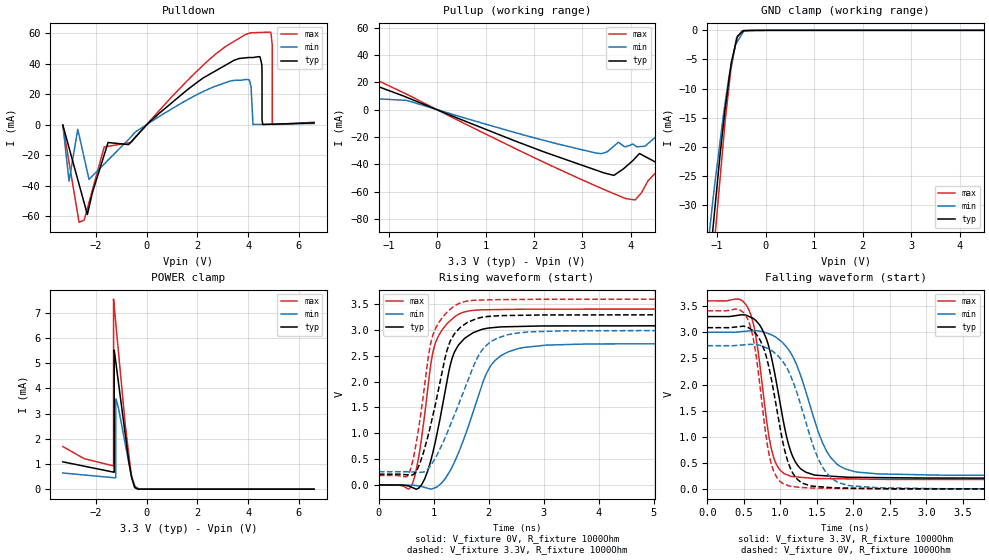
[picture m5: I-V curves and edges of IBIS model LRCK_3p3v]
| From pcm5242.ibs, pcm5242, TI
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|   Model
[Model]   LRCK_3p3v
Model_type   I/O
Polarity   Non-Inverting
Enable   Active-Low
Vinl = 0.99
Vinh = 2.31
Vmeas = 1.65
Vref = 0
Cref = 1pF
Rref = 1000000
|   typ   min   max
C_comp   1.193pF   1.163pF   1.236pF
[Voltage Range]   3.3   3   3.6
[Temperature Range]   27   105   -25
[Pullup Reference]   3.3   3   3.6
[Pulldown Reference]   -0   -0   -0
[Power Clamp Reference]   3.3   3   3.6
[GND Clamp Reference]   -0   -0   -0
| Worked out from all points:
|   slope of the pulldown table from 0 to 0.495 V, typ, clamps not added: 64.7 ohm
|   slope of the pullup table from 0 to 0.495 V, typ, clamps not added: 69.1 ohm
|   GND clamp passes 1 mA (typ) near -0.58 V on its own axis
|   POWER clamp passes 1 mA (typ) near -0.68 V on its own axis
|   falling waveform, V_fixture 3.3V, R_fixture 1000Ohm: 20-80 % time 269ps typ, 407ps min, 199ps max; typ from 3.3 V to 0.207 V
|   rising waveform, V_fixture 0V, R_fixture 1000Ohm: 20-80 % time 359ps typ, 556ps min, 277ps max; typ from 0 V to 3.09 V
|   rising waveform, V_fixture 3.3V, R_fixture 1000Ohm: 20-80 % time 401ps typ, 626ps min, 299ps max; typ from 0.207 V to 3.3 V
|   falling waveform, V_fixture 0V, R_fixture 1000Ohm: 20-80 % time 264ps typ, 397ps min, 195ps max; typ from 3.09 V to 0 V
[Pulldown]
|   Voltage   I(typ)   I(min)   I(max)
-3.3V     -378.6uA   -354.3uA   -383.8uA
-3.055V   -15.23mA   -37.15mA   -24.72mA
-2.66V    -39.19mA   -6.88mA    -64mA
-2.269V   -54.26mA   -35.93mA   -51.02mA
-1.518V   -11.76mA   -23.31mA   -14.25mA
3.893V    43.72mA    29.58mA    58.97mA
4.473V    44.3mA     92.29uA    60.35mA
4.899V    184uA      218.7uA    60.28mA
4.952V    211.8uA    234.3uA    51.71mA
4.954V    212.8uA    234.8uA    45.96mA
4.954V    213uA      234.9uA    123.7nA
6.6V      1.085mA    722.9uA    1.49mA
[GND Clamp]
|   Voltage   I(typ)   I(min)   I(max)
-3.3V     -526.5mA   -489.6mA   -552.8mA
-1.164V   -40.81mA   -35.07mA   -48.1mA
-1.079V   -33.47mA   -28.6mA    -39.08mA
-1.046V   -30.55mA   -26.19mA   -35.49mA
-940.1mV  -21.43mA   -19.22mA   -25.56mA
-837.1mV  -13.61mA   -12.6mA    -15.87mA
-718mV    -6.168mA   -6.453mA   -6.856mA
-600.4mV  -1.708mA   -2.193mA   -1.374mA
-580.8mV  -1.006mA   -1.922mA   -1.157mA
-482.7mV  -273.3uA   -561.9uA   -69.67uA
-284.5mV  -34uA      -2.302uA   -308.8nA
6.6V      0A         0A         0A
[Pullup]
|   Voltage   I(typ)   I(min)   I(max)
-3.3V     20.89mA    12mA       56.35mA
-2.931V   39.44mA    11.28mA    50.14mA
3.451V    -46.27mA   -31.45mA   -58.41mA
4.087V    -35.4mA    -26.27mA   -65.94mA
4.851V    -29.44mA   -9.628mA   -42.22mA
5.092V    -17.54mA   16.01mA    -44.35mA
5.643V    53.42mA    42.85mA    12.66mA
5.844V    57.49mA    46.25mA    45.19mA
6.411V    39.73mA    55.8mA     58.85mA
6.425V    38.25mA    56.04mA    20.59mA
6.504V    29.88mA    -235.4mA   -195.5mA
6.6V      -527.7mA   -587.8mA   -456.8mA
[POWER Clamp]
|   Voltage   I(typ)   I(min)   I(max)
-3.3V     1.085mA    641.9uA    1.693mA
-1.306V   677.2uA    455.6uA    924.8uA
-1.303V   676.5uA    455.2uA    1.01mA
-1.303V   676.5uA    455.2uA    1.69mA
-1.303V   676.4uA    455.2uA    7.179mA
-1.303V   676.4uA    455.2uA    7.549mA
-1.276V   766.2uA    452.7uA    7.258mA
-1.276V   5.221mA    452.7uA    7.257mA
-1.275V   5.526mA    452.7uA    7.255mA
-1.206V   4.992mA    3.578mA    6.509mA
-482.7mV  140.9uA    192.3uA    79.12uA
6.6V      0A         0A         0A
[Ramp]
R_load = 1000
|   typ   min   max
dV/dt_r   1.85276/3.58741e-10   1.64632/5.53781e-10   2.04618/2.76561e-10
dV/dt_f   1.85579/2.6927e-10   1.64679/4.06983e-10   2.05064/1.98632e-10
[Falling Waveform]
V_fixture = 3.3V
V_fixture_min = 3V
V_fixture_max = 3.6V
R_fixture = 1000Ohm
C_fixture = 0F
|   Time   V(typ)   V(min)   V(max)
0s        3.3V       3V         3.6V
565.5ps   3.304V     3.025V     3.437V
675.7ps   3.206V     3.028V     2.818V
830ps     2.78V      2.977V     1.126V
894.2ps   2.411V     2.94V      671.4mV
1.141ns   727.9mV    2.607V     246.7mV
1.287ns   380.2mV    2.135V     226.4mV
1.631ns   253.8mV    730.7mV    201.1mV
2.023ns   226mV      334.4mV    194.4mV
10ns      207mV      255.4mV    182.3mV
[Rising Waveform]
V_fixture = 0V
V_fixture_min = 0V
V_fixture_max = 0V
R_fixture = 1000Ohm
C_fixture = 0F
|   Time   V(typ)   V(min)   V(max)
0s        1.762nV    46.88nV    912.6pV
565.5ps   -31.63mV   -4.28mV    -62.7mV
779.9ps   6.321mV    -32.44mV   929.2mV
939.8ps   450.6mV    -79.6mV    2.294V
1.029ns   844.6mV    -52.35mV   2.748V
1.312ns   2.372V     304.1mV    3.193V
1.544ns   2.821V     883.5mV    3.347V
2.023ns   3.042V     2.288V     3.394V
2.57ns    3.069V     2.648V     3.403V
10ns      3.088V     2.744V     3.41V
[Rising Waveform]
V_fixture = 3.3V
V_fixture_min = 3V
V_fixture_max = 3.6V
R_fixture = 1000Ohm
C_fixture = 0F
|   Time   V(typ)   V(min)   V(max)
0s        207mV      255.3mV    182.3mV
513.1ps   196mV      255mV      165.5mV
679.1ps   265.1mV    247.5mV    806.9mV
917ps     1.047V     339.7mV    2.594V
985.5ps   1.359V     446.3mV    2.911V
1.287ns   2.754V     1.123V     3.392V
1.544ns   3.098V     1.813V     3.547V
1.933ns   3.256V     2.681V     3.584V
2.513ns   3.284V     2.941V     3.592V
10ns      3.3V       3V         3.6V
[Falling Waveform]
|Gnd
V_fixture = 0V
V_fixture_min = 0V
V_fixture_max = 0V
R_fixture = 1000Ohm
C_fixture = 0F
|   Time   V(typ)   V(min)   V(max)
0s        3.088V     2.744V     3.41V
553.7ps   3.093V     2.765V     3.245V
653.7ps   2.99V      2.764V     2.681V
792.8ps   2.601V     2.711V     1.122V
871.3ps   2.139V     2.657V     502.7mV
1.109ns   498.7mV    2.263V     65.91mV
1.268ns   146.3mV    1.662V     34mV
1.574ns   43.03mV    427.5mV    18.81mV
1.947ns   19.52mV    68.33mV    11.79mV
10ns      6.649uV    68.74uV    2.391uV
